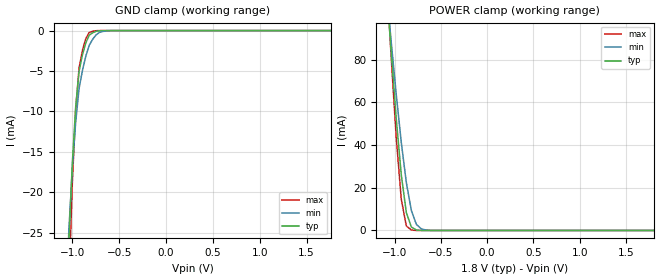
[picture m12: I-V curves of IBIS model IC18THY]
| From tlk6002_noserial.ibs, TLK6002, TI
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[Model]   IC18THY
Model_type   Input
Polarity   Non-Inverting
Vinl =  0.63
Vinh =  1.17
C_comp   0.6387869p   0.5480567p   0.7549689p
[Model Spec]
Vinl   0.63   0.5985   0.6615
Vinh   1.17   1.1115   1.2285
[Temperature Range]   25   125   -40
[Voltage Range]   1.8   1.71   1.89
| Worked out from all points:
|   GND clamp passes 1 mA (typ) near -0.84 V on its own axis
|   POWER clamp passes 1 mA (typ) near -0.79 V on its own axis
[POWER_clamp]
-1.8V     607mA      492.8mA    733.5mA
-1.055V   94.75mA    97.21mA    95.13mA
-1.036V   83.56mA    88.51mA    81.22mA
-981.8mV  52.51mA    63.81mA    43.47mA
-927.3mV  26.09mA    41.33mA    14.63mA
-872.7mV  8.397mA    22.47mA    2.133mA
-818.2mV  1.587mA    9.312mA    180.8uA
-763.6mV  228.2uA    2.824mA    13.3uA
-709.1mV  29.94uA    699uA      954.2nA
-654.5mV  3.826uA    158.9uA    68.5nA
1.8V      3.537pA    1.47pA     16.11pA
[GND_clamp]
-1.8V     -539.1mA   -380.2mA   -748.9mA
-1.036V   -26.23mA   -24.68mA   -32.15mA
-1V       -16.52mA   -17.21mA   -19.02mA
-963.6mV  -9.451mA   -11.37mA   -9.842mA
-927.3mV  -5.032mA   -7.151mA   -4.619mA
-890.9mV  -2.977mA   -4.906mA   -2.412mA
-854.5mV  -1.487mA   -3.125mA   -949uA
-818.2mV  -563.1uA   -1.808mA   -231uA
-781.8mV  -269.9uA   -1.064mA   -91.3uA
-709.1mV  -19.12uA   -213.6uA   -1.453uA
-600mV    -278.7nA   -13.18uA   -6.862nA
1.764V    3.096pA    9.108pA    10.16pA
